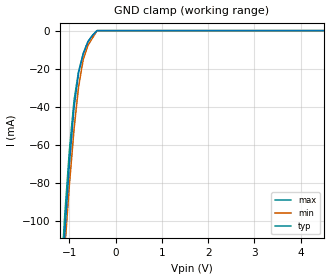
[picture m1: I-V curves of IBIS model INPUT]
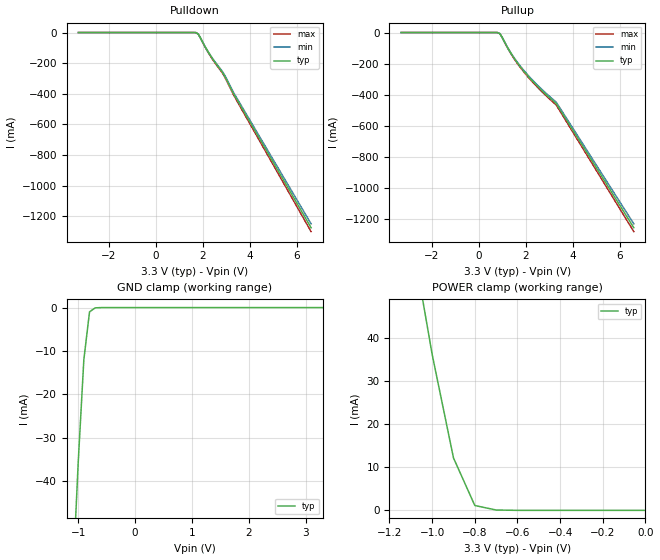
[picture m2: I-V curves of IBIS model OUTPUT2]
|   PERICOM SEMICONDUCTOR CORP
|   IBIS Model of PI6C4911506-06
|   Product Family: 6C
|   TSSOP Package 24 Pin (L)
[IBIS Ver] 3.2
[Comment char] |_char
[File Name] pi6c4911506-06.ibs
[File Rev] 2.0
[Source] File originated at Pericom Semiconductor Corp.
[Date] 02/01/2015
[Disclaimer] (C) Copyright PERICOM Semiconductor Corporation
   All rights reserved
  Pericom Semiconductor Corporation hereby grants the user of
  this IBIS model a non-exclusive, nontransferable license to
  use this IBIS model under the following terms.
  This IBIS model is provided on an "AS IS" basis and Pericom
  makes absolutely no warranty with respect to the information
  contained herein. PERICOM DISCLAIMS AND CUSTOMER WAIVES ALL
  WARRANTIES, EXPRESSED OR IMPLIED, INCLUDING WARRANTIES OF
  MERCHANTABILITY OR FITNESS FOR A PARTICULAR PURPOSE. The
  entire risk as to quality and performance is with the customer.
  Accordingly, in no event shall the company be liable for any
  damages, whether in contract or tort, including any lost
  profits or other incidental, consequential, exemplary, or
  punitive damages arising out of the use or application of the
  IBIS model provided in this package. Further, Pericom reserves
  the right to make changes without notice to any product herein
  to improve reliability, function, or design. Pericom does not
  convey any license under patent rights or any other intellectual
  property rights, including those of third parties.
  The user is granted this license only to use the IBIS model
  and is not granted rights to sell, load, rent, lease or license
  the IBIS model in whole or in part, or in modified form to anyone
  other than user. User may modify the IBIS model to suit its specific
  application but rights to derivative works and such modifications
  shall belong to Pericom.
  Pericom is not obligated to provide maintenance or support
  for the licensed IBIS model.
  Contact Pericom at ATTN: APPLICATIONS ENGINEERING / IBIS MODELS
  3545 North first street, San Jose, CA 95134
[Component] pi6c4911506-06
[Manufacturer] Pericom Semiconductor Corp.
[Package]
| variable   typ   min  max
R_pkg   0.03869ohm   NA   NA
L_pkg   2.64482nH   NA   NA
C_pkg   0.19279pF   NA   NA
[Pin]   signal_name   model_name   R_pin   L_pin   C_pin
1   nQ2   OUTPUT2   0.04069   3.22001nH   0.23014pF
2   Q2   OUTPUT2   0.03969   2.93241nH   0.21146pF
3   VDD   POWER   0.03869   2.64482nH   0.19279pF
4   nQ1   OUTPUT2   0.04069   3.22001nH   0.23014pF
5   Q1   OUTPUT2   0.03969   2.93241nH   0.21146pF
6   VEE   GND   0.04069   3.22001nH   0.23014pF
7   nQ0   OUTPUT2   0.04069   3.22001nH   0.23014pF
8   Q0   OUTPUT2   0.03969   2.93241nH   0.21146pF
9   CLK_SEL0   INPUT   0.03768   2.35722nH   0.17411pF
10   XTAL_IN   INPUT   0.03768   2.35722nH   0.17411pF
|11   XTAL_OUT   OUTPUT   0.03768   2.35722nH   0.17411pF
12   CLK_EN   INPUT   0.03768   2.35722nH   0.17411pF
13   CLK0   INPUT   0.03768   2.35722nH   0.17411pF
14   CLK1   INPUT   0.03768   2.35722nH   0.17411pF
15   nCLK1   INPUT   0.03768   2.35722nH   0.17411pF
16   CLK_SEL1   INPUT   0.03768   2.35722nH   0.17411pF
17   nQ5   OUTPUT2   0.04069   3.22001nH   0.23014pF
18   Q5   OUTPUT2   0.03969   2.93241nH   0.21146pF
19   VDD   POWER   0.03869   2.64482nH   0.19279pF
20   nQ4   OUTPUT2   0.04069   3.22001nH   0.23014pF
21   Q4   OUTPUT2   0.03969   2.93241nH   0.21146pF
22   VDD   POWER   0.03869   2.64482nH   0.19279pF
23   nQ3   OUTPUT2   0.04069   3.22001nH   0.23014pF
24   Q3   OUTPUT2   0.03969   2.93241nH   0.21146pF
[Diff Pin]  inv_pin vdiff   tdelay_typ tdelay_min tdelay_max
2   1   NA   0ns   -0.05ns   0.05ns
5   4   NA   0ns   -0.05ns   0.05ns
8   7   NA   0ns   -0.05ns   0.05ns
18   17   NA   0ns   -0.05ns   0.05ns
21   20   NA   0ns   -0.05ns   0.05ns
24   23   NA   0ns   -0.05ns   0.05ns
| Models and submodels in the file (2): INPUT (Input), OUTPUT2 (Output_ECL)
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|   Model INPUT
[Model] INPUT
Model_type Input
Vinl = 800mV
Vinh = 2.00V
| variable   typ   min   max
C_comp   4.00pF   3.8pF   4.2pF
[Voltage Range]   3.30V   3.0V   3.6V
[GND Clamp Reference]   0.00V   0.00V   0.00V
[POWER Clamp Reference]  3.30V   3.0V   3.6V
[temperature range]   25   85   -40
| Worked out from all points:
|   GND clamp passes 1 mA (typ) near -0.44 V on its own axis
[GND Clamp]
| Voltage   I(typ)   I(min)   I(max)
-3.3V     -1.197A    -928.6mA   -1.231A
-1.202V   -148.7mA   -152.6mA   -137.9mA
-1.101V   -107.3mA   -115.3mA   -97.36mA
-999.4mV  -69.97mA   -80.92mA   -62.79mA
-898.4mV  -40.31mA   -51.53mA   -36.54mA
-802.2mV  -22.43mA   -29.68mA   -21.51mA
-701mV    -12.09mA   -15.2mA    -12.13mA
-599.9mV  -5.88mA    -7.79mA    -5.84mA
-498.6mV  -2.39mA    -3.78mA    -2.44mA
-402.8mV  0A         0A         0A
6.601V    30uA       0A         0A
[POWER Clamp]   |Note: Vtable = Vcc - Voutput
| Voltage   I(typ)   I(min)   I(max)
-3.3V     0A         0A         0A
0V        0A         0A         0A
| Model  OUTPUT2 (PECL)
[Model]  OUTPUT2
Model_type  Output_ECL
Polarity Non-Inverting
Enable Active-High
Vmeas = 1.975V | Vmeas = ( VOH - VOL ) / 2 + VOL
Rref = 50.0
Cref = 0
Vref = 1.3V | Vref = vcc - 2V
C_comp   2pF   1.5pF   2.5pF
[Voltage Range]   3.30V   3.00V   3.60V
| Open source, no load
[POWER Clamp Reference]   3.30V   3.00V   3.60V
[Pullup Reference]   3.30V   3.00V   3.60V
[Pulldown Reference]   3.30V   3.00V   3.60V
[GND Clamp Reference]   0.00V   0.00V   0.00V
[temperature range]   25   85   -40
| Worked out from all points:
|   GND clamp passes 1 mA (typ) near -0.80 V on its own axis
|   POWER clamp passes 1 mA (typ) near -0.79 V on its own axis
[GND_clamp]
| voltage = voutput
| voltage   I(typ)   I(min)   I(max)
-3.3V     -1.04A     NA         NA
-1.1V     -64.4mA    NA         NA
-1V       -35.9mA    NA         NA
-900mV    -12mA      NA         NA
-800mV    -978uA     NA         NA
-700mV    -63.5uA    NA         NA
3.3V      13.2pA     NA         NA
[POWER_clamp]
| voltage = vcc - voutput
| voltage   I(typ)   I(min)   I(max)
-3.3V     783mA      NA         NA
-1.1V     64.9mA     NA         NA
-1V       36.3mA     NA         NA
-900mV    12.2mA     NA         NA
-800mV    1.13mA     NA         NA
-700mV    81.2uA     NA         NA
0V        13.2pA     NA         NA
[Pulldown]
| voltage = vcc - voutput
| voltage   I(typ)   I(min)   I(max)
-3.3V     0A         0A         0A
1.6V      -12.23uA   -11.01uA   -13.45uA
1.7V      -542.5uA   -488.2uA   -596.7uA
1.8V      -10.52mA   -10.31mA   -10.73mA
2.3V      -147.2mA   -144.3mA   -150.1mA
2.9V      -277.8mA   -272.2mA   -283.4mA
3.3V      -399.5mA   -391.5mA   -407.5mA
6.6V      -1.275A    -1.25A     -1.3A
[Pullup]
| voltage = vcc -voutput
| voltage   I(typ)   I(min)   I(max)
-3.3V     0A         0A         0A
700mV     -5.881uA   -5.293uA   -6.469uA
900mV     -6.916mA   -6.778mA   -7.054mA
1.4V      -140.7mA   -137.9mA   -143.5mA
1.9V      -245mA     -240.1mA   -249.9mA
2.5V      -345.4mA   -338.5mA   -352.3mA
3.3V      -457.6mA   -448.4mA   -466.8mA
6.6V      -1.257A    -1.232A    -1.282A
[Ramp]
| variable typ   min   max
dV/dt_r 450m/244.42p   450m/268.862p   450m/219.978p
dV/dt_f 450m/195.22p   450m/214.742p   450m/175.698p
R_load = 50.00
